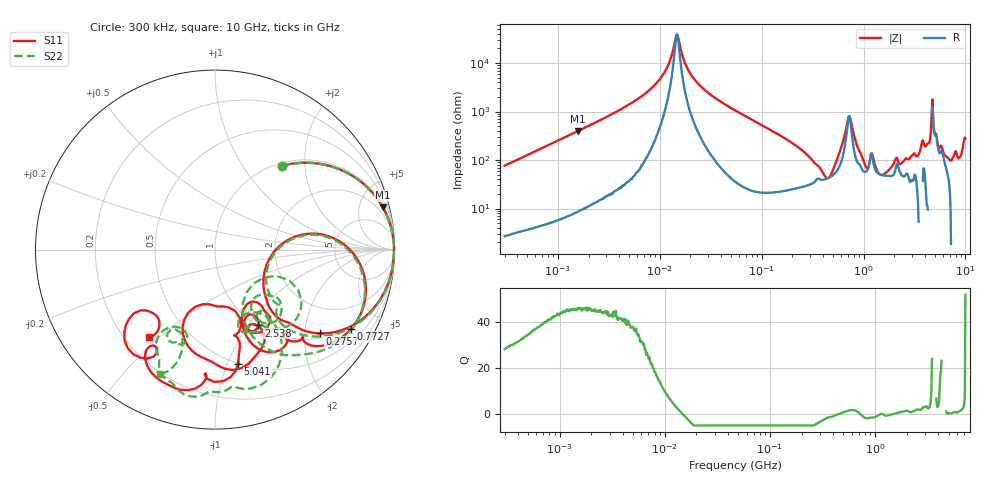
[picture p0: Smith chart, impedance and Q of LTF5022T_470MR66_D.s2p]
! S-Parameter Data Generated by TDK Corporation
! Copyright(C) 2020 TDK Corporation.
! All Rights Reserved.
! TDK P/N: LTF5022T-470MR66-D (Inductor)
! Property: L=47uH at 100kHz
! Size(LxWxT): 6.5x5x2.2mm
! Model Type: s2p (Touchstone File Format Version 1.0)
! Frequency: DC=Yes Start=0.3MHz Stop=10000MHz 802points Log-sweep
! Model Generated on Apr. 23, 2020
! Port Assignments:
!  1 ---@@@--- 2
! Applicable Conditions:
!  Temperature = 25 degC
!  DC Bias Current = 0 A
!  Small Signal Operation
! Terms and conditions regarding TDK Simulation Models
! (1)This simulation model is being provided solely for informational purposes. Please refer to the specifications of the products in terms of detailed characteristics of such products.
! (2)In no event shall TDK Corporation of any of its subsidiaries be liable for any loss or damage arising, directly or indirectly,
!  From any information contained in this simulation model, including, but not limited to loss or damages arising from any inaccuracies, omissions or errors in connection with such information.
! (3)Any and all copyrights on this simulation model are owned by TDK Corporation.
!  Duplication or redistribution of this simulation model without prior written permission from TDK Corporation is prohibited.
! (4)This simulation model is subject to any modification or change without any prior notice.
! (5)Neither TDK Corporation nor any of its subsidiaries shall make any warranty, express or implied,
!  Including but not limited to the correctness, implied warranties of merchantability and fitness for a particular purpose with respect to this simulation models.
! (6)The use of this simulation model shall be deemed to have consented to the terms and conditions hereof.
# Hz S MA R 50
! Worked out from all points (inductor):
!   801 points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, 300 kHz to 10 GHz, reference 50 ohm
!   read as one part in series: L = 40.2 uH near 318.3 kHz
!   highest Q = 46.1 at 1.574 MHz (marker M1), where L = 40 uH
!   self-resonance near 14.71 MHz
!   S11 on the Smith chart (normalised r, x): 300 kHz: 1.05, +1.52; 275.7 MHz: 1.13, -2.38; 772.7 MHz: 0.91, -3.49; 2.538 GHz: 1.01, -1.12; 5.041 GHz: 0.49, -1.09; 10 GHz: 0.30, -0.46
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300000  0.5963 51.4  0.7823 -36.5  0.7821 -36.5  0.5957 51.4
1573603  0.9643 14.1  0.244 -74.7  0.2439 -74.7  0.9644 14.1
1713600  0.9693 12.9  0.2248 -75.8  0.2249 -75.8  0.9693 12.9
9671944  0.9976 1.1  0.02352 -83.8  0.02352 -83.8  0.9975 1.0
1.470778e7  0.9974 -0.4  0.002572 -5.9  0.00257 -6.0  0.9973 -0.5
2.220835e7  0.9969 -1.9  0.02256 81.3  0.02257 81.4  0.997 -2.0
5.477226e7  0.9924 -6.9  0.09346 81.0  0.09347 81.0  0.9923 -7.1
2.756623e8  0.7467 -38.7  0.5291 38.0  0.5292 38.0  0.737 -41.1
3.126428e8  0.6585 -42.7  0.5888 28.2  0.5889 28.2  0.631 -46.5
4.568044e8  0.2999 -21.1  0.693 -10.0  0.693 -10.0  0.3095 -19.5
5.497689e8  0.5272 9.6  0.5636 -39.9  0.5636 -40.0  0.5332 8.9
7.152593e8  0.8833 -19.5  0.11 -30.8  0.11 -30.8  0.8832 -21.1
7.726947e8  0.8775 -30.2  0.1692 21.2  0.1691 21.2  0.8765 -32.2
1.054047e9  0.6189 -51.7  0.5394 -5.7  0.5395 -5.7  0.4617 -67.7
1.228555e9  0.6414 -63.0  0.4032 -8.3  0.4031 -8.3  0.5866 -35.8
1.767019e9  0.3558 -54.8  0.6166 -52.6  0.6163 -52.6  0.3479 -51.0
2.53795e9  0.4868 -60.2  0.4925 -94.8  0.4919 -94.8  0.4803 -52.1
3.640519e9  0.5335 -108.4  0.2116 -154.7  0.2105 -154.6  0.7018 -58.2
4.107799e9  0.3178 -86.8  0.1859 -137.6  0.1872 -137.6  0.7719 -83.4
5.040844e9  0.652 -78.6  0.0969 -99.9  0.09739 -100.2  0.7763 -109.1
6.899057e9  0.7209 -122.6  0.2045 -150.5  0.2045 -151.0  0.562 -109.9
1e10  0.6081 -127.1  0.07028 103.1  0.07046 102.2  0.76 -113.9
